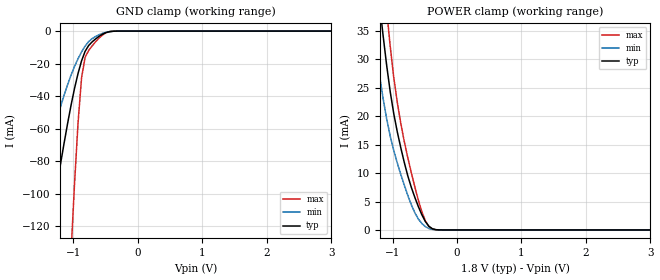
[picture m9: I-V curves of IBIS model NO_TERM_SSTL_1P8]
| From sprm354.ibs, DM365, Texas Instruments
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|   Model Cell NO_TERM_SSTL_1P8
|NO_TERM_SSTL_1P8
[Model]   NO_TERM_SSTL_1P8
Model_type   Input
Polarity   Non-Inverting
Vinl =  0.8
Vinh =  1
C_comp   3.009089p   2.23501p   3.950269p
[Model Spec]
Vinl   0.8   0.71   0.89
Vinh   1   0.91   1.09
[Temperature Range]   25   125   -40
[Voltage Range]   1.8   1.62   1.98
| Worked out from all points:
|   GND clamp passes 1 mA (typ) near -0.50 V on its own axis
|   POWER clamp passes 1 mA (typ) near -0.46 V on its own axis
[POWER_clamp]
|   voltage   I(typ)   I(min)   I(max)
-1.8V     107.1mA    82.38mA    134mA
-1.309V   51.28mA    36.03mA    66.97mA
-1.145V   34.1mA     23.06mA    45.37mA
-1.091V   28.94mA    19.52mA    38.61mA
-1.036V   24.34mA    16.53mA    32.34mA
-981.8mV  20.5mA     14.01mA    26.9mA
-818.2mV  11.9mA     7.885mA    15.55mA
-654.5mV  5.743mA    3.031mA    7.577mA
-490.9mV  1.486mA    587.8uA    1.604mA
-381.8mV  216.1uA    94.9uA     155.6uA
-272.7mV  11.41uA    9.679uA    3.89uA
3.545V    0A         0A         0A
[GND_clamp]
|   voltage   I(typ)   I(min)   I(max)
-1.8V     -229.3mA   -132mA     -818.5mA
-1.745V   -215.8mA   -124mA     -769.6mA
-1.691V   -202.2mA   -116mA     -720.6mA
-1.364V   -121.3mA   -68.84mA   -424.9mA
-1.036V   -45.75mA   -27.16mA   -136.8mA
-981.8mV  -35.29mA   -21.77mA   -94.06mA
-927.3mV  -26.08mA   -17mA      -56.49mA
-872.7mV  -18.32mA   -12.82mA   -28.79mA
-818.2mV  -12.5mA    -9.274mA   -16.24mA
-654.5mV  -4.818mA   -3.298mA   -6.568mA
-381.8mV  -101.4uA   -119.6uA   -85.85uA
3.545V    0A         0A         0A
